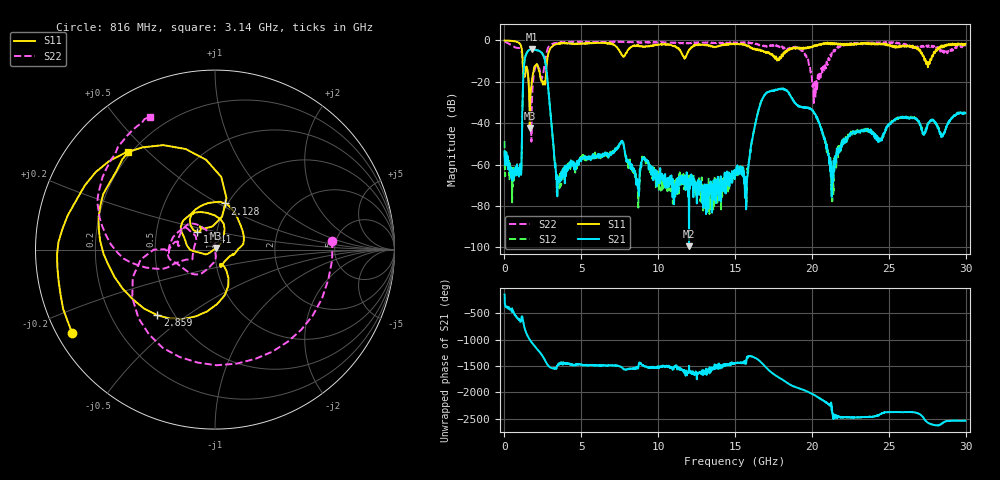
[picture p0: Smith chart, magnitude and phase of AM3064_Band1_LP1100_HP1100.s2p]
# Hz S DB R 50.0
!freq dBS11 angS11 dBS21 angS21 dBS12 angS12 dBS22 angS22
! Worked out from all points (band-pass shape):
!   1600 points, 10 MHz to 29.98 GHz, reference 50 ohm
!   highest |S21| = -4.21 dB at 1.791 GHz (marker M1); lowest = -99.4 dB at 12.01 GHz (marker M2)
!   |S21| within 3 dB of the highest: 1.384 GHz to 2.527 GHz (1.143 GHz wide, 58.5 % of centre)
!   lowest |S11| = -42.4 dB at 1.641 GHz (marker M3), VSWR 1.02, Z = 50.4 + j0.635 ohm
!   |S11| at or under -10 dB: 1.186 GHz to 2.771 GHz (1.585 GHz wide, 80.1 % of centre); 27.4 GHz to 27.68 GHz (282.7 MHz wide, 1.03 % of centre)
!   |S22| runs from -48.9 to -0.5 dB; largest |S21 - S12| = 0.011
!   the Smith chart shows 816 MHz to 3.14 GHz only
!   S11 on the Smith chart (normalised r, x): 816 MHz: 0.04, -0.27; 1.341 GHz: 0.81, +0.16; 2.128 GHz: 0.97, +0.54; 2.859 GHz: 0.41, -0.39; 3.14 GHz: 0.19, +0.43
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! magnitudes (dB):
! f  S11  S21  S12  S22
! 10 MHz  -0.1  -53.5  -48.6  -0.5
! 816 MHz  -0.7  -59.9  -60.0  -3.7
! 1.022 GHz  -1.8  -59.7  -62.4  -3.9
! 1.341 GHz  -17.2  -8.3  -8.3  -14.0
! 1.641 GHz  -42.4  -4.5  -4.5  -25.1
! 1.791 GHz  -19.5  -4.2  -4.2  -28.4
! 2.128 GHz  -11.6  -4.8  -4.8  -11.9
! 2.859 GHz  -6.3  -24.0  -24.0  -3.3
! 3.14 GHz  -2.8  -47.1  -47.4  -1.7
! 3.553 GHz  -1.6  -68.0  -66.9  -1.2
! 5.015 GHz  -1.6  -57.1  -55.7  -0.7
! 7.62 GHz  -7.0  -48.7  -48.5  -0.7
! 8.632 GHz  -2.7  -67.7  -70.7  -1.0
! 10 GHz  -2.1  -69.0  -66.7  -0.9
! 12.01 GHz  -4.7  -99.4  -71.5  -1.4
! 15 GHz  -1.9  -65.2  -64.4  -1.4
! 15.74 GHz  -2.4  -79.9  -78.2  -1.2
! 17.05 GHz  -5.8  -25.4  -25.3  -3.2
! 19.99 GHz  -3.4  -33.4  -33.5  -17.7
! 21.28 GHz  -1.6  -75.5  -68.1  -6.2
! 25 GHz  -2.0  -40.9  -40.5  -1.2
! 29.98 GHz  -1.7  -35.1  -35.2  -2.9
